(* Logix 5000 AddOnInstructionDefinition export CIP_Axis_Disable; software revision 34.01; part 4 of 4 *)
(* tags used below, declared in another part *)
   Axis : CIP_Axis;
(* CIP_Drive_Comms_Single_Axis, continued *)

ROUTINE Prescan   (* ladder *)
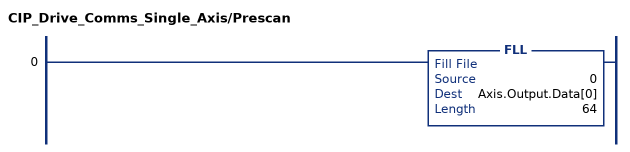
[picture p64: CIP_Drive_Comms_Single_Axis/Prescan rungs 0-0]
   0: FLL(0,Axis.Output.Data[0],64);
END_ROUTINE
END_ADD_ON_INSTRUCTION
